FUNCTION "Traslazione pallet" : VOID
TITLE =
VERSION : 0.1
//KNOW_HOW_PROTECT

VAR_TEMP
  Error_block_move : INT ;
END_VAR
BEGIN
NETWORK
TITLE =

NETWORK
TITLE =Traslazione dati a postazione 2 per traslazione pallet
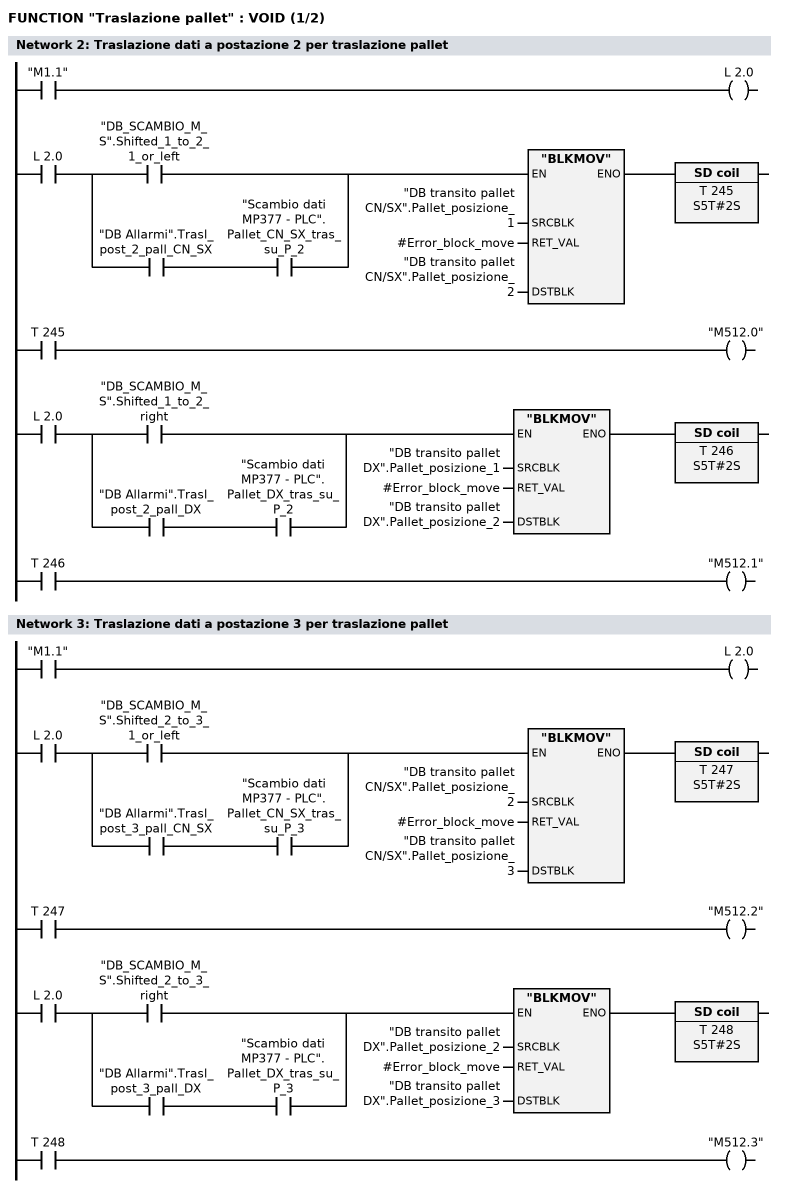
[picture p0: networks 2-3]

      U     "M1.1";
      =     L      2.0;
      U(    ;
      U     L      2.0;
      U(    ;
      O     "DB_SCAMBIO_M_S".Shifted_1_to_2_1_or_left;
      O     ;
      U     "DB Allarmi".Trasl_post_2_pall_CN_SX;
      U     "Scambio dati MP377 - PLC".Pallet_CN_SX_tras_su_P_2;
      )     ;
      SPBNB _001;
      CALL "BLKMOV" (
           SRCBLK                   := "DB transito pallet CN/SX".Pallet_posizione_1,
           RET_VAL                  := #Error_block_move,
           DSTBLK                   := "DB transito pallet CN/SX".Pallet_posizione_2);
_001: U     BIE;
      )     ;
      L     S5T#2S;
      SE    T    245;
      NOP   0;
      NOP   0;
      NOP   0;
      U     T    245;
      =     "M512.0";
      U(    ;
      U     L      2.0;
      U(    ;
      O     "DB_SCAMBIO_M_S".Shifted_1_to_2_right;
      O     ;
      U     "DB Allarmi".Trasl_post_2_pall_DX;
      U     "Scambio dati MP377 - PLC".Pallet_DX_tras_su_P_2;
      )     ;
      SPBNB _002;
      CALL "BLKMOV" (
           SRCBLK                   := "DB transito pallet DX".Pallet_posizione_1,
           RET_VAL                  := #Error_block_move,
           DSTBLK                   := "DB transito pallet DX".Pallet_posizione_2);
_002: U     BIE;
      )     ;
      L     S5T#2S;
      SE    T    246;
      NOP   0;
      NOP   0;
      NOP   0;
      U     T    246;
      =     "M512.1";
NETWORK
TITLE =Traslazione dati a postazione 3 per traslazione pallet

      U     "M1.1";
      =     L      2.0;
      U(    ;
      U     L      2.0;
      U(    ;
      O     "DB_SCAMBIO_M_S".Shifted_2_to_3_1_or_left;
      O     ;
      U     "DB Allarmi".Trasl_post_3_pall_CN_SX;
      U     "Scambio dati MP377 - PLC".Pallet_CN_SX_tras_su_P_3;
      )     ;
      SPBNB _003;
      CALL "BLKMOV" (
           SRCBLK                   := "DB transito pallet CN/SX".Pallet_posizione_2,
           RET_VAL                  := #Error_block_move,
           DSTBLK                   := "DB transito pallet CN/SX".Pallet_posizione_3);
_003: U     BIE;
      )     ;
      L     S5T#2S;
      SE    T    247;
      NOP   0;
      NOP   0;
      NOP   0;
      U     T    247;
      =     "M512.2";
      U(    ;
      U     L      2.0;
      U(    ;
      O     "DB_SCAMBIO_M_S".Shifted_2_to_3_right;
      O     ;
      U     "DB Allarmi".Trasl_post_3_pall_DX;
      U     "Scambio dati MP377 - PLC".Pallet_DX_tras_su_P_3;
      )     ;
      SPBNB _004;
      CALL "BLKMOV" (
           SRCBLK                   := "DB transito pallet DX".Pallet_posizione_2,
           RET_VAL                  := #Error_block_move,
           DSTBLK                   := "DB transito pallet DX".Pallet_posizione_3);
_004: U     BIE;
      )     ;
      L     S5T#2S;
      SE    T    248;
      NOP   0;
      NOP   0;
      NOP   0;
      U     T    248;
      =     "M512.3";
NETWORK
TITLE =Traslazione dati a postazione 4 per traslazione pallet
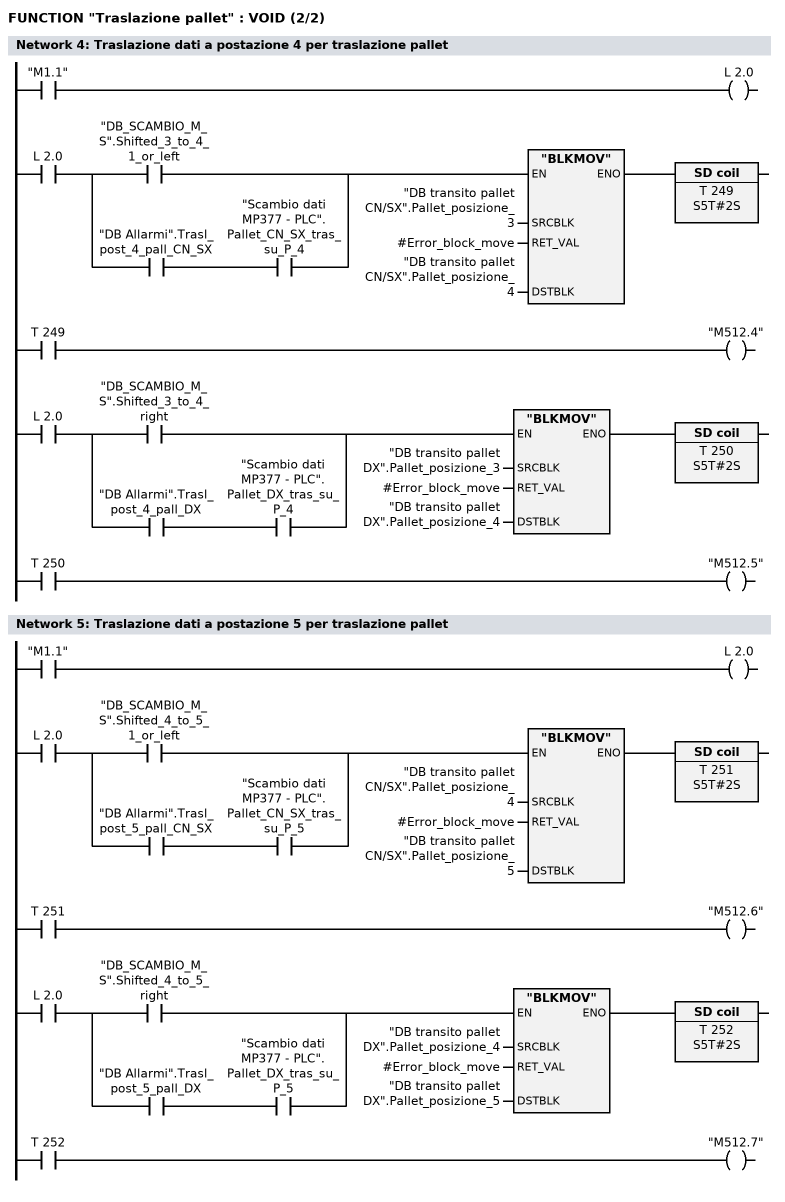
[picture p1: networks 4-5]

      U     "M1.1";
      =     L      2.0;
      U(    ;
      U     L      2.0;
      U(    ;
      O     "DB_SCAMBIO_M_S".Shifted_3_to_4_1_or_left;
      O     ;
      U     "DB Allarmi".Trasl_post_4_pall_CN_SX;
      U     "Scambio dati MP377 - PLC".Pallet_CN_SX_tras_su_P_4;
      )     ;
      SPBNB _005;
      CALL "BLKMOV" (
           SRCBLK                   := "DB transito pallet CN/SX".Pallet_posizione_3,
           RET_VAL                  := #Error_block_move,
           DSTBLK                   := "DB transito pallet CN/SX".Pallet_posizione_4);
_005: U     BIE;
      )     ;
      L     S5T#2S;
      SE    T    249;
      NOP   0;
      NOP   0;
      NOP   0;
      U     T    249;
      =     "M512.4";
      U(    ;
      U     L      2.0;
      U(    ;
      O     "DB_SCAMBIO_M_S".Shifted_3_to_4_right;
      O     ;
      U     "DB Allarmi".Trasl_post_4_pall_DX;
      U     "Scambio dati MP377 - PLC".Pallet_DX_tras_su_P_4;
      )     ;
      SPBNB _006;
      CALL "BLKMOV" (
           SRCBLK                   := "DB transito pallet DX".Pallet_posizione_3,
           RET_VAL                  := #Error_block_move,
           DSTBLK                   := "DB transito pallet DX".Pallet_posizione_4);
_006: U     BIE;
      )     ;
      L     S5T#2S;
      SE    T    250;
      NOP   0;
      NOP   0;
      NOP   0;
      U     T    250;
      =     "M512.5";
NETWORK
TITLE =Traslazione dati a postazione 5 per traslazione pallet

      U     "M1.1";
      =     L      2.0;
      U(    ;
      U     L      2.0;
      U(    ;
      O     "DB_SCAMBIO_M_S".Shifted_4_to_5_1_or_left;
      O     ;
      U     "DB Allarmi".Trasl_post_5_pall_CN_SX;
      U     "Scambio dati MP377 - PLC".Pallet_CN_SX_tras_su_P_5;
      )     ;
      SPBNB _007;
      CALL "BLKMOV" (
           SRCBLK                   := "DB transito pallet CN/SX".Pallet_posizione_4,
           RET_VAL                  := #Error_block_move,
           DSTBLK                   := "DB transito pallet CN/SX".Pallet_posizione_5);
_007: U     BIE;
      )     ;
      L     S5T#2S;
      SE    T    251;
      NOP   0;
      NOP   0;
      NOP   0;
      U     T    251;
      =     "M512.6";
      U(    ;
      U     L      2.0;
      U(    ;
      O     "DB_SCAMBIO_M_S".Shifted_4_to_5_right;
      O     ;
      U     "DB Allarmi".Trasl_post_5_pall_DX;
      U     "Scambio dati MP377 - PLC".Pallet_DX_tras_su_P_5;
      )     ;
      SPBNB _008;
      CALL "BLKMOV" (
           SRCBLK                   := "DB transito pallet DX".Pallet_posizione_4,
           RET_VAL                  := #Error_block_move,
           DSTBLK                   := "DB transito pallet DX".Pallet_posizione_5);
_008: U     BIE;
      )     ;
      L     S5T#2S;
      SE    T    252;
      NOP   0;
      NOP   0;
      NOP   0;
      U     T    252;
      =     "M512.7";
END_FUNCTION

